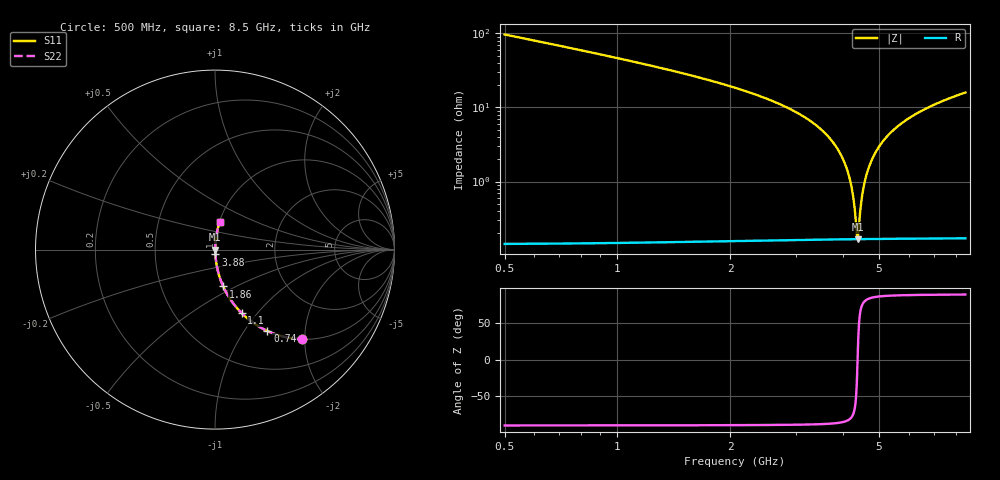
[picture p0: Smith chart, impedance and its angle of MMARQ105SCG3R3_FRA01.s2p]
! MMARQ105SCG3R3_FRA01  S-PARAMETER MODEL  ( General Type )
! Model Generated by TAIYO YUDEN Corporation (http://www.ty-top.com)
! Version 1.0
! TAIYO YUDEN Control No. 200326
! Copyright(c) 2020 TAIYO YUDEN CO.,LTD. All Rights Reserved.
! Product Description (link to TY-COMPAS)
! https://ds.yuden.co.jp/TYCOMPAS/or/detail?pn=MMARQ105SCG3R3BFRA01&u=M
! Products Name : Multilayer Ceramic Capacitors
! Characteristics :
!  Capacitance : 3.3 pF , Rated Voltage : 250V , TCC : CG / C0G
!  Case Size : 1.0 x 0.5 / 0.039 x 0.02 [mm/inch] , Thickness : 0.5 / 0.02 [mm/inch]
!  (Conditions: Temperature = 25 degC , DC Bias Current/Voltage = 0A / 0V)
! External Node Assignments :
!  1  o---| |---o  2
! GND o---------o GND
! Frequency Range : 500MHz  -  8.5GHz  [ 401 STEP ]
# MHz S RI R 50
! Freq[MHz].  S11 Real  S11 Imag  S21 Real  S21 Imag  S12 Real  S12 Imag  S22 Real  S22 Imag
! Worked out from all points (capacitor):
!   401 points, 500 MHz to 8.5 GHz, reference 50 ohm
!   read as one part in series: C = 3.26 pF near 540 MHz
!   lowest |Z| = 167 mohm at 4.38 GHz (marker M1)
!   series resonance near 4.38 GHz, so ESL is about 410 pH
!   S11 on the Smith chart (normalised r, x): 500 MHz: 1.00, -1.93; 740 MHz: 1.00, -1.28; 1.1 GHz: 1.00, -0.83; 1.86 GHz: 1.00, -0.43; 3.88 GHz: 1.00, -0.05; 8.5 GHz: 1.00, +0.32
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500  0.4822 -0.4989  0.5178 0.4989  0.5178 0.4989  0.4822 -0.4989
740  0.2921 -0.4536  0.7079 0.4536  0.7079 0.4536  0.2921 -0.4536
1100  0.1486 -0.3539  0.8514 0.3539  0.8514 0.3539  0.1486 -0.3539
1840  0.047 -0.2081  0.953 0.2081  0.953 0.2081  0.047 -0.2081
1860  0.0457 -0.2052  0.9543 0.2052  0.9543 0.2052  0.0457 -0.2052
3180  0.00686 -0.072  0.9931 0.072  0.9931 0.072  0.00686 -0.072
3580  0.00369 -0.0451  0.9963 0.0451  0.9963 0.0451  0.00369 -0.0451
3880  0.00239 -0.027  0.9976 0.027  0.9976 0.027  0.00239 -0.027
4060  0.00195 -0.0169  0.9981 0.0169  0.9981 0.0169  0.00195 -0.0169
4180  0.00177 -0.0104  0.9982 0.0104  0.9982 0.0104  0.00177 -0.0104
4260  0.0017 -0.0062  0.9983 0.0062  0.9983 0.0062  0.0017 -0.0062
4340  0.00167 -0.00206  0.9983 0.00206  0.9983 0.00206  0.00167 -0.00206
4380  0.00167 -2.21e-05  0.9983 2.21e-05  0.9983 2.21e-05  0.00167 -2.21e-05
4420  0.00167 0.002  0.9983 -0.002  0.9983 -0.002  0.00167 0.002
4500  0.00171 0.00599  0.9983 -0.00599  0.9983 -0.00599  0.00171 0.00599
4560  0.00175 0.00893  0.9982 -0.00893  0.9982 -0.00893  0.00175 0.00893
4660  0.00186 0.0138  0.9981 -0.0138  0.9981 -0.0138  0.00186 0.0138
4920  0.00235 0.0259  0.9977 -0.0259  0.9977 -0.0259  0.00235 0.0259
5300  0.0035 0.0425  0.9965 -0.0425  0.9965 -0.0425  0.0035 0.0425
5840  0.00588 0.0645  0.9941 -0.0645  0.9941 -0.0645  0.00588 0.0645
7180  0.0146 0.1129  0.9854 -0.1129  0.9854 -0.1129  0.0146 0.1129
8500  0.0262 0.1545  0.9738 -0.1545  0.9738 -0.1545  0.0262 0.1545
